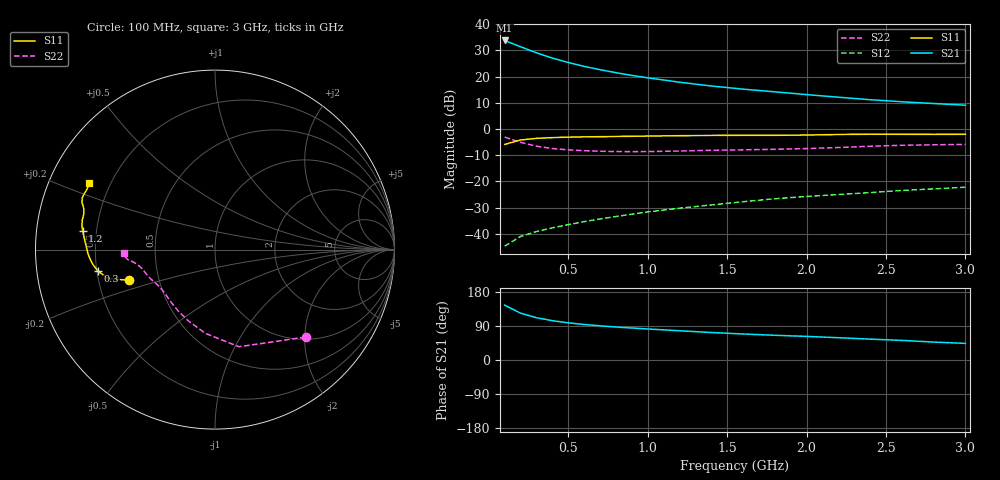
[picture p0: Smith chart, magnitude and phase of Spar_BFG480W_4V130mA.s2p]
! Filename: 4130BFG480.001
! Title: BFG480W
! Bias: Vce=4V; Ic=130mA
! Company: NXP Semiconductors NL
! User: Quality&Reliability T&D
! Measure time: 10 Nov 1999 / 12:04:37
#  MHz  S  MA  R 50
! Freq  S11  S21  S12  S22  :
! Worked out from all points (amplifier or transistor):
!   20 points, 100 MHz to 3 GHz, reference 50 ohm
!   highest |S21| = 33.8 dB at 100 MHz (marker M1)
!   |S21| within 3 dB of that: start of sweep to 226.5 MHz
!   unconditionally stable (mu >= 1): 586.1 MHz to end of sweep
!   at 400 MHz: K = 0.89, MSG = 32.4 dB, |S12| = -37.7 dB
!   at 1.2 GHz: K = 1.10, MAG = 22.1 dB, |S12| = -30.2 dB
!   at 3 GHz: K = 1.06, MAG = 14.2 dB, |S12| = -22.2 dB
!   S11 on the Smith chart (normalised r, x): 100 MHz: 0.34, -0.15; 300 MHz: 0.20, -0.09; 1.2 GHz: 0.15, +0.07; 3 GHz: 0.12, +0.24
100  0.5076 -160.3  48.75 144.7  0.005832 68.0  0.7018 -44.0
200  0.6171 -164.9  37.03 123.6  0.008926 60.9  0.5574 -76.1
300  0.6622 -169.5  28.39 111.7  0.01108 60.9  0.4696 -96.6
400  0.685 -173.0  22.52 103.8  0.01304 63.4  0.4244 -110.4
500  0.6984 -175.8  18.54 98.1  0.01499 65.7  0.4 -120.3
600  0.708 -178.1  15.65 93.7  0.01712 67.6  0.3858 -127.5
700  0.7134 179.9  13.52 90.2  0.01926 69.6  0.3768 -133.0
800  0.7198 178.0  11.85 87.1  0.02142 71.3  0.3717 -137.6
900  0.726 176.2  10.53 84.4  0.0237 73.0  0.3698 -141.6
1000  0.7326 174.7  9.463 81.9  0.02619 73.9  0.3711 -145.2
1200  0.7452 171.8  7.805 77.2  0.03088 75.2  0.3805 -150.9
1400  0.7538 169.6  6.602 72.5  0.03561 76.1  0.3925 -155.1
1600  0.7576 167.2  5.756 68.6  0.04105 76.6  0.4005 -158.4
1800  0.7573 164.7  5.115 65.2  0.04676 76.9  0.4096 -161.9
2000  0.7664 162.6  4.526 62.3  0.05162 77.3  0.4232 -166.2
2200  0.7856 160.6  4.038 58.8  0.05624 77.2  0.4434 -169.7
2400  0.7938 158.8  3.616 55.1  0.06121 76.6  0.4686 -172.0
2600  0.7924 157.1  3.302 51.7  0.06742 75.9  0.489 -173.4
2800  0.7883 154.8  3.06 47.3  0.07217 74.4  0.4996 -175.2
3000  0.7931 152.1  2.841 43.9  0.07761 73.5  0.5083 -178.0
